PROGRAM MAIN
VAR
	eComState 				: E_ComState;
	
	(* slave *)
	AODB					: ARRAY[0..1] OF ST_IEC870_5_101AODBEntry; // Application object data base
	hServer					: T_HSERVER;
	fbSlave					: FB_IEC870_5_104Slave;	
	
	fbValueManipTime		: TON;			// time for value manipulation - example
END_VAR

CASE eComState OF
INIT:
// INIT slave
	// TCP/IP server handle
	F_CreateServerHnd( 	'', 			// own (slave) TwinCAT netID, empty string = local
						'127.0.0.1',	// own (slave) IP address
						2404,			//communication port - check firewall settings
						LISTEN_MODE_CLOSEALL OR CONNECT_MODE_ENABLEDBG, // close all previous opened socket connections and enable debug output
						TRUE,			// enable connection
						hServer );			

	// system parameter					
	fbSlave.sysPara.asduAddr 	:= 3;  	// common ASDU address
	fbSlave.sysPara.dbgMode 	:= IEC870_DEBUGMODE_DEVSTATE  OR IEC870_DEBUGMODE_LINKERROR;(*OR IEC870_DEBUGMODE_ASDU OR IEC870_DEBUGMODE_LINKLAYER*);(* enable output of device state change messages *)


// INIT data points
	// SLAVE -> MASTER (monitoring direction)
		
		(* bSlaveToMaster - single point in monitoring direction *)
		F_iecInitAOEntry( 	M_SP_NA_1,			// type is single point
							10,					// information object address
							IEC870_GRP_INROGEN, // general interrogation group and spontaneous data transmission
							0,					// multiplier - not used 
							MAP_AREA_MEMORY,	// map this datapoint FROM PLC by address
							0,					// map FROM byte offset		AT%MX0.0 -> 0 byte offset
							0,					// map FROM bit offset		AT%MX0.0 -> 0 bit offset
							AODB[0] );			//data base array element
						
						
	//MASTER -> SLAVE (control directon)	
	
		(* bMasterToSlave - single point in command direction *)
		F_iecInitAOEntry(	C_SC_NA_1,			// type is single command
							101, 				// information object address
							0,  				// group - not used
							0, 					// multiplier - not used 
							MAP_AREA_MEMORY, 	// map this datapoint TO PLC memory area (buffer)
							5, 					// map TO byte offset		AT%MX5.0 -> 5 byte offset
							0, 					// map TO bit offset		AT%MX5.0 -> 0 bit offset
							AODB[1] );			// data base array element
									
			
	eComState := COMMUNICATION;
		
COMMUNICATION:	// INIT completed
	
	(* execute IEC slave function block *)
	fbSlave( bEnable 	:= TRUE,
			hServer 	:= hServer, 		// server connection handle
			pAOEntries 	:= ADR(AODB),
			cbAOEntries := SIZEOF(AODB),		
			pInputs 	:= 0,				// intput buffer where the data point values are mapped to and from
			cbInputs	:= 0,				(* not used in this example project *)
			pOutputs 	:= 0,				// output buffer where the data point values are mapped to and from
			cbOutputs 	:= 0,				(* not used in this example project *)	
			pMemory 	:= ADR(memory),		// memory buffer where the data point values are mapped to and from
			cbMemory 	:= SIZEOF(memory),
			pData 		:= 0,				// data buffer where the data point values are mapped to and from
			cbData 		:= 0 );				(* not used in this example project *)
			
			
	(* Check for device errors, remove them and log message to the TwinCAT System Manager log view *)
	REPEAT
		fbSlave.system.device.errors.RemoveError();
		IF fbSlave.system.device.errors.bOk THEN
			ADSLOGSTR( ADSLOG_MSGTYPE_ERROR OR ADSLOG_MSGTYPE_LOG, 'IEC60870-5-104 slave error: 0x%s',
						DWORD_TO_HEXSTR( fbSlave.system.device.errors.getError.nErrId, 8, FALSE) );
		END_IF
	UNTIL NOT fbSlave.system.device.errors.bOk
	END_REPEAT

END_CASE


// bSlaveToMaster value manipulation
fbValueManipTime(IN:= NOT fbValueManipTime.Q, PT:= T#1S);
IF fbValueManipTime.Q THEN
	bSlaveToMaster := NOT bSlaveToMaster;
END_IF

END_PROGRAM
